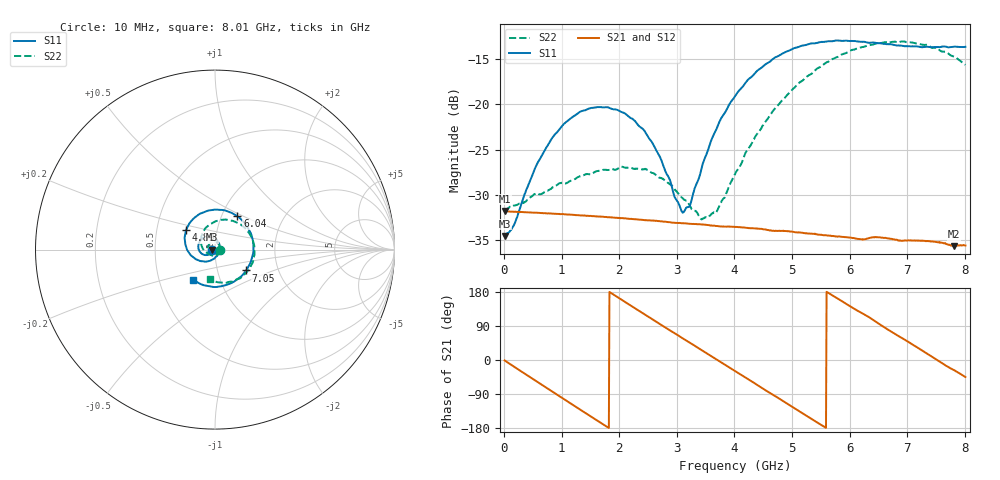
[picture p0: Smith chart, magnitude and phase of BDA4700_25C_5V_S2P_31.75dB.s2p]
!Agilent Technologies,E5071B,MY42404982,A.09.10
!Date: Mon Oct 20 13:42:38 2025
!Data & Calibration Information:
!Freq	S11:SOLT2(ON)	S21:SOLT2(ON)	S12:SOLT2(ON)	S22:SOLT2(ON)
# Hz S RI R 50
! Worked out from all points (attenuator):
!   801 points, 10 MHz to 8.01 GHz, reference 50 ohm
!   highest |S21| = -31.80 dB at 20 MHz (marker M1); lowest = -35.7 dB at 7.81 GHz (marker M2)
!   lowest |S11| = -34.5 dB at 10 MHz (marker M3), VSWR 1.04, Z = 48.2 - j0.0873 ohm
!   |S11| at or under -10 dB: start of sweep to end of sweep
!   |S22| runs from -32.7 to -13.1 dB; largest |S21 - S12| = 0.00021
!   S11 on the Smith chart (normalised r, x): 10 MHz: 0.96, -0.00; 4.89 GHz: 0.71, +0.16; 6.04 GHz: 1.19, +0.46; 7.05 GHz: 1.37, -0.33; 8.01 GHz: 0.74, -0.26
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1e7  -0.0187 -0.000906  0.0257 -0.000539  0.0257 -0.000578  0.0263 -0.000821
2e7  -0.019 -0.00143  0.0257 -0.000951  0.0256 -0.000989  0.0262 -0.00109
1.6e8  -0.0192 -0.00879  0.0245 -0.00715  0.0245 -0.00712  0.0264 -0.00757
5.5e8  -0.0353 -0.028  0.0145 -0.0206  0.0145 -0.0206  0.0154 -0.0282
8.1e8  -0.0554 -0.0304  0.00408 -0.0246  0.00406 -0.0246  -0.00185 -0.034
1.35e9  -0.0918 0.00214  -0.0168 -0.0176  -0.0168 -0.0176  -0.036 -0.0178
2.09e9  -0.0551 0.0702  -0.0211 0.0101  -0.0211 0.0102  -0.0294 0.0338
2.68e9  0.012 0.0516  -0.00291 0.0224  -0.00291 0.0224  0.0126 0.0375
2.97e9  0.0261 0.0156  0.00762 0.0208  0.00764 0.0207  0.0254 0.0219
3.13e9  0.0247 -0.00695  0.0128 0.0179  0.0128 0.0179  0.0282 0.00922
3.24e9  0.0189 -0.0211  0.0157 0.0153  0.0157 0.0152  0.027 0.0015
3.54e9  -0.0118 -0.0544  0.0207 0.00578  0.0208 0.00565  0.0131 -0.0199
3.7e9  -0.0376 -0.0642  0.0213 0.000126  0.0213 7.96e-05  -0.000464 -0.0259
4.01e9  -0.0934 -0.0593  0.0184 -0.0101  0.0184 -0.0101  -0.032 -0.0257
4.89e9  -0.1601 0.1107  -0.00769 -0.0184  -0.00764 -0.0184  -0.0733 0.0821
5.35e9  -0.0774 0.2025  -0.0177 -0.00767  -0.0177 -0.00773  -0.0155 0.1473
6.04e9  0.1249 0.1858  -0.0137 0.0121  -0.0138 0.012  0.139 0.1432
6.68e9  0.2148 0.00275  0.00353 0.0178  0.00358 0.0178  0.2196 0.000486
7.05e9  0.1741 -0.116  0.0125 0.0125  0.0126 0.0124  0.1967 -0.0981
7.46e9  0.0601 -0.198  0.0173 0.00173  0.0173 0.00172  0.1113 -0.1723
7.81e9  -0.0611 -0.1987  0.0147 -0.00738  0.0148 -0.00742  0.0182 -0.1826
8.01e9  -0.1227 -0.1677  0.0117 -0.0117  0.0118 -0.0118  -0.0297 -0.1623
